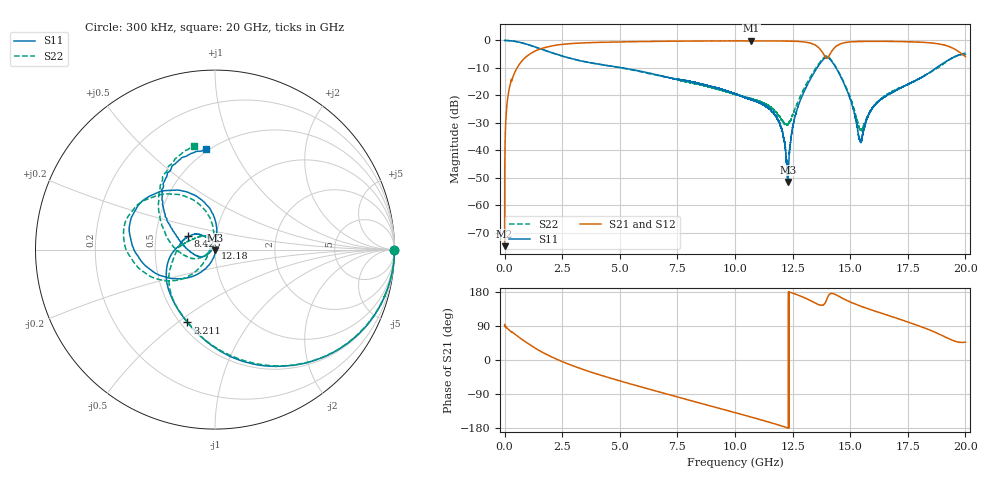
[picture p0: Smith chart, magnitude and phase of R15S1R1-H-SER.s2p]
!{R15S1R1}
!Johanson Technology Inc.
!www.johansontechnology.com
!Test Board Conditions:
!Substrate Type  RO4350B
!Substrate Thickness  20 mil
!Substrate Dk  3.66
!TL Type: GCPW
!TL Trace Width  34 mil
!TL Gap  10 mil
!Electrode orientation  Horizontal
!DUT TOPOLOGY	SERIES
!Mounting Pad LxW  26x52 mil
! Created Sat Feb  6 12:11:15 2021
# hz S ma R 50
! 2 Port Network Data from SP1.SP block
! freq  magS11  angS11  magS21  angS21  magS12  angS12  magS22  angS22
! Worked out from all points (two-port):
!   20001 points, 300 kHz to 20 GHz, reference 50 ohm
!   highest |S21| = -0.13 dB at 10.71 GHz (marker M1); lowest = -74.8 dB at 300 kHz (marker M2)
!   |S21| within 3 dB of the highest: 1.535 GHz to 13.69 GHz (12.15 GHz wide, 160 % of centre); 14.27 GHz to 19.53 GHz (5.261 GHz wide, 31.1 % of centre)
!   lowest |S11| = -51.5 dB at 12.3 GHz (marker M3), VSWR 1.01, Z = 50.2 - j0.155 ohm
!   |S11| at or under -10 dB: 5.13523 GHz to 5.13705 GHz (1.82 MHz wide, 0.0354 % of centre); 5.14 GHz to 13.56 GHz (8.418 GHz wide, 90 % of centre); 14.38 GHz to 18.74 GHz (4.357 GHz wide, 26.3 % of centre)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
!   |S22| runs from -32.9 to 0.0 dB; largest |S21 - S12| = 0.012
!   S11 on the Smith chart (normalised r, x): 300 kHz: open; 3.211 GHz: 0.54, -0.54; 8.425 GHz: 0.73, +0.11; 12.18 GHz: 1.00, +0.02; 20 GHz: 0.49, +0.79
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300000  0.9976 -0.1  0.0001811 93.7  0.000236 83.2  0.9964 -0.2
1.323e8  0.9956 -7.0  0.08789 82.7  0.08843 82.7  0.9955 -7.0
4.983e8  0.9548 -24.0  0.293 65.8  0.294 65.9  0.9535 -23.8
1.8693e9  0.6359 -76.8  0.7658 13.3  0.7675 13.3  0.6328 -76.2
3.2113e9  0.4339 -110.8  0.8935 -20.7  0.8948 -20.8  0.4347 -110.2
3.3343e9  0.4228 -113.4  0.8982 -23.4  0.8993 -23.4  0.4233 -112.9
6.6673e9  0.2336 -176.9  0.9626 -83.6  0.9638 -83.6  0.2295 -170.5
8.4253e9  0.1664 153.6  0.9779 -112.9  0.9767 -112.9  0.1595 163.6
1.00003e10  0.1073 132.1  0.9823 -138.9  0.9829 -138.9  0.1048 134.9
1.07093e10  0.08389 123.6  0.9852 -150.7  0.9813 -150.8  0.08685 119.4
1.17313e10  0.04348 97.9  0.9799 -168.7  0.9804 -168.7  0.05106 117.9
1.21783e10  0.01117 76.6  0.9759 -177.0  0.9761 -177.1  0.03045 153.3
1.23023e10  0.002651 -35.6  0.9741 -179.7  0.973 -179.5  0.03031 178.9
1.26513e10  0.04817 -100.8  0.9644 173.1  0.965 173.1  0.06358 -136.1
1.33343e10  0.2216 -134.6  0.8781 155.1  0.8807 155.0  0.2402 -137.9
1.38943e10  0.4748 172.3  0.5185 148.4  0.5188 148.1  0.5017 177.8
1.41873e10  0.4206 128.4  0.626 175.7  0.6269 175.3  0.4369 135.7
1.49423e10  0.09993 83.9  0.9369 154.6  0.9329 154.6  0.1072 94.4
1.54453e10  0.01466 149.0  0.9623 142.4  0.9591 142.3  0.0239 148.2
1.66673e10  0.1046 -160.7  0.9638 117.2  0.9549 117.2  0.1077 -152.8
1.84163e10  0.2586 155.9  0.9076 80.0  0.9045 79.8  0.2534 170.7
2e10  0.5578 94.6  0.5087 47.2  0.5025 47.3  0.5883 100.9
